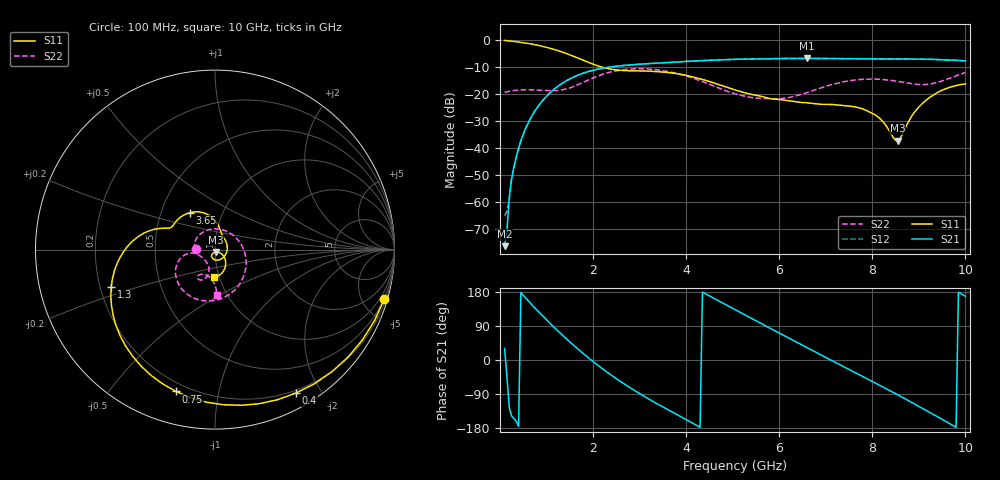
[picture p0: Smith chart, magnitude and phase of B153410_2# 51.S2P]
!  2-Port S-parameters saved by WinCal
! VAR MeasName=S-Parameters (CALIBRATED_DATA) read from VNA (N5245A)
! VAR MeasDate=2016-12-23 10:02:03
! VAR NAME=B153410_2# 51
! VAR FILENAME=B153410_2# 51.S2P
! VAR DATE=2016-12-23 10:02:03
! VAR PHYS_PORTS=1,2
# Hz S DB R 50
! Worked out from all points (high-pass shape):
!   199 points, 100 MHz to 10 GHz, reference 50 ohm
!   highest |S21| = -6.79 dB at 6.6 GHz (marker M1); lowest = -76.2 dB at 100 MHz (marker M2)
!   |S21| within 3 dB of the highest: 2.45 GHz to end of sweep
!   lowest |S11| = -37.2 dB at 8.55 GHz (marker M3), VSWR 1.03, Z = 50.4 - j1.33 ohm
!   |S11| at or under -10 dB: 2.191 GHz to end of sweep
!   |S22| runs from -21.8 to -10.6 dB; largest |S21 - S12| = 0.0022
!   S11 on the Smith chart (normalised r, x): 100 MHz: 0.45, -7.02; 400 MHz: 0.17, -1.70; 750 MHz: 0.16, -0.75; 1.3 GHz: 0.25, -0.17; 3.65 GHz: 0.70, +0.31; 10 GHz: 0.95, -0.30
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1e8  -0.16 -16.2  -76.23 30.6  -64.90 3.2  -19.38 179.5
1.5e8  -0.23 -23.9  -70.53 -43.5  -63.52 -41.3  -19.16 177.3
2e8  -0.33 -31.5  -58.22 -125.8  -59.28 -112.9  -18.95 174.5
2.5e8  -0.42 -39.0  -51.56 -147.6  -50.84 -145.6  -18.85 172.1
4e8  -0.75 -60.5  -39.87 -175.2  -40.28 -172.3  -18.49 162.9
7.5e8  -1.73 -105.3  -26.26 137.3  -26.25 137.9  -18.47 134.9
1e9  -2.69 -132.6  -20.82 105.7  -20.78 106.0  -18.67 108.6
1.3e9  -4.22 -160.1  -16.44 70.2  -16.41 70.2  -18.55 67.4
1.75e9  -7.19 170.8  -12.50 21.0  -12.50 20.9  -15.96 0.3
2.6e9  -11.21 153.4  -9.50 -57.5  -9.50 -57.6  -11.09 -86.5
3.4e9  -11.67 133.4  -8.52 -117.0  -8.53 -117.1  -11.09 -136.9
3.65e9  -12.09 124.2  -8.26 -134.1  -8.27 -134.2  -11.79 -148.8
4.35e9  -14.56 97.5  -7.59 179.2  -7.60 179.2  -15.35 -170.0
5.05e9  -18.44 77.5  -7.12 132.8  -7.15 132.9  -19.87 -165.0
5.85e9  -21.76 54.7  -6.89 80.9  -6.90 81.1  -21.74 -136.4
6.6e9  -23.23 3.8  -6.79 32.6  -6.81 32.7  -19.41 -108.5
6.7e9  -23.43 -4.9  -6.80 26.2  -6.81 26.2  -18.83 -107.1
7.75e9  -25.24 -98.1  -6.97 -40.8  -6.94 -40.6  -14.57 -114.5
8.35e9  -33.10 -118.8  -7.02 -79.2  -7.00 -79.0  -14.81 -122.4
8.55e9  -37.17 -72.2  -7.00 -92.1  -7.00 -92.1  -15.30 -122.9
9.1e9  -23.07 -40.4  -7.09 -129.0  -7.09 -128.9  -16.48 -109.8
1e10  -16.20 -91.2  -7.71 168.3  -7.71 168.5  -12.00 -87.8
